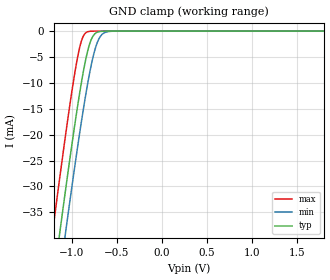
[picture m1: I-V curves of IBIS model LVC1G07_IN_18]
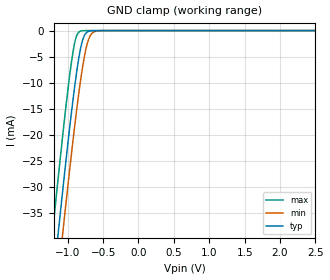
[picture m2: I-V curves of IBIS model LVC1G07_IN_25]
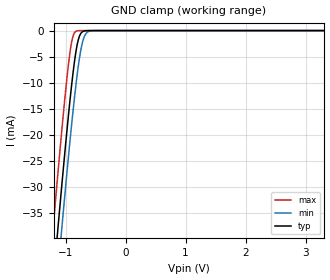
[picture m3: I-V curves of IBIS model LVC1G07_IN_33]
| TEXAS INSTRUMENTS INCORPORATED
| Standard Linear and Logic Group
| IBIS Model of SN74LVC1G07
| SINGLE BUFFER/DRIVER WITH OPEN-DRAIN OUTPUT
| This file contains package information for the following:
|  SON 6-pin (DSF) package as [Component] LVC1G07_DSF
|  SOT 5-pin (DBV) package as [Component] LVC1G07_DBV
|  SOT 5-pin (DCK) package as [Component] LVC1G07_DCK
|  NanoStar WCSP 5-pin (YEP) package as [Component] LVC1G07_YEP
|  NanoFree WCSP 5-pin (YZP) package as [Component] LVC1G07_YZP
|  NanoFree WCSP 5-pin (YZT) package as [Component] LVC1G07_YZT
| This device can be powered at the following Vccs:
|  1.8 volt Vcc
|  2.5 volt Vcc
|  3.3 volt Vcc
|  5 volt Vcc
| This file provides unique models under the [Model Selector] for each Vcc.
| For operation at a specific Vcc, select the appropriate model after each
| [Model Selector] keyword.
[IBIS Ver]   3.2
[Comment char]  |_char
[File Name]   sn74lvc1g07.ibs
[File Rev]   1.4 | d_die
[Date]   03/06/2014
[Source]
| Texas Instruments Incorporated.
| Analog-eLab Design Center, HPA
| 12500 TI Blvd
| Dallas, TX -75243
[Notes]   Revision History:
| The following is an IBIS list for the SN74LVC1G07.
| Please contact sllibis@ti.com with questions and
| comments concerning SLL IBIS models.
| - FILE REV HISTORY
| - 1.2 YEP and YZP packages added on 10/15/2004
| - 1.3 YZT package added on 02/23/2005
| - Power clamp data deleted as there is no power-clamp diode.
| - The slow Rising Waveforms in the LVC1G07_OUT are normal for
|   this open-drain (TPLZ) device.
| - 1.4 DSF package added 03/06/2014.
[Disclaimer]
| Property of Texas Instruments Incorporated.  Unauthorized
| reproduction and/or distribution is strictly prohibited.
| This product is protected under copyright law.
| Created  2002, (C) Copyright  2002, Texas Instruments
| Incorporated, All Rights Reserved
| UNLESS THERE IS A SIGNED, WRITTEN AGREEMENT TO THE
| CONTRARY, TEXAS INSTRUMENTS (TI) IS PROVIDING THE IBIS
| MODELS  AND WITHOUT ANY WARRANTY, EXPRESSED OR
| IMPLIED.  TI assumes no liability for:
|  1) the accuracy of the IBIS models provided to your
|   company;
|  2) the proper functioning of these IBIS Models in your
|   design or for any resulting applications; or
|  3) infringement of patents, copyrights or intellectual
|   property rights resulting from your use of these IBIS
|   models.
| TI provides IBIS Models as a service to our customers.
| You and your company shall not distribute, sell or give
| these models to anyone else without prior written
| permission from TI.
| TI reserves the right to make changes to our products or
| to discontinue any semiconductor product or service
| without notice, and advises our customers to obtain the
| latest version of relevant information to verify, before
| placing orders, that the information being relied on is
| current.
| Please be aware that your receipt and use of the IBIS
| information provided shall serve as acceptance of these
| terms and conditions.  If you do not accept these terms,
| you should return or destroy the IBIS models and any
| other accompanying information immediately.
[Copyright]
(C) Copyright 2014 Texas Instruments Incorporated.All rights reserved.
| Component LVC1G07_DSF 6-pin SON
[Component]   LVC1G07_DSF
[Manufacturer]   Texas Instruments, Inc.
[Package]
|   typ   min   max
R_pkg   0.041145   0.03325   0.04904
L_pkg   0.422435nH  0.33414nH   0.51073nH
C_pkg   0.109645pF  0.10407pF   0.11522pF
[Pin]   signal_name   model_name   R_pin   L_pin   C_pin
1   nc   nc   0.00109   0.02796nH   0.07413pF
2   A   LVC1G07_IN   0.03325   0.33414nH   0.10407pF
3   GND   GND   0.04429   0.45885nH   0.11133pF
4   Y   LVC1G07_OUT   0.04904   0.51073nH   0.11522pF
5   nc   nc   0.00037   0.03788nH   0.07652pF
6   VCC   POWER   0.04377   0.44894nH   0.11085pF
| Component LVC1G07_DBV 5-pin SOT
[Component]   LVC1G07_DBV
[Manufacturer]   Texas Instruments, Inc.
[Package]
|   typ   min   max
R_pkg   2.500e-02   2.100e-02   2.900e-02
L_pkg   1.529e-09   1.312e-09   1.906e-09
C_pkg   1.560e-13   1.100e-13   2.400e-13
[Pin]   signal_name   model_name   R_pin   L_pin   C_pin
1   NC   NC   2.100e-02   1.511e-09   1.440e-13
2   A   LVC1G07_IN   2.300e-02   1.312e-09   1.380e-13
3   GND   GND   2.900e-02   1.906e-09   2.400e-13
4   Y   LVC1G07_OUT   2.600e-02   1.541e-09   1.500e-13
5   VCC   POWER   2.500e-02   1.374e-09   1.100e-13
| Component LVC1G07_DCK 5-pin SOT
[Component]   LVC1G07_DCK
[Manufacturer]   Texas Instruments, Inc.
[Package]
|   typ   min   max
R_pkg   2.000e-02   1.700e-02   2.500e-02
L_pkg   9.980e-10   8.810e-10   1.069e-09
C_pkg   1.460e-13   1.180e-13   2.050e-13
[Pin]   signal_name   model_name   R_pin   L_pin   C_pin
1   NC   NC   1.900e-02   1.069e-09   1.620e-13
2   A   LVC1G07_IN   1.800e-02   8.810e-10   1.210e-13
3   GND   GND   1.700e-02   1.031e-09   2.050e-13
4   Y   LVC1G07_OUT   2.000e-02   9.600e-10   1.240e-13
5   VCC   POWER   2.500e-02   1.049e-09   1.180e-13
| Component LVC1G07_YEP 5-pin NanoStar WCSP
[Component]   LVC1G07_YEP
[Manufacturer]   Texas Instruments, Inc.
[Package]
|   typ   min   max
R_pkg   0.001   0.001   0.001
L_pkg   0.021nH   0.021nH   0.021nH
C_pkg   0.046pF   0.045pF   0.047pF
[Pin]   signal_name   model_name   R_pin   L_pin   C_pin
1   DNU   LVC1G07_IN   0.001   0.021nH   0.046pF
2   A   LVC1G07_IN   0.001   0.021nH   0.047pF
3   GND   GND   0.001   0.021nH   0.046pF
4   Y   LVC1G07_OUT   0.001   0.021nH   0.045pF
5   VCC   POWER   0.001   0.021nH   0.045pF
| Component LVC1G07_YZP 5-pin NanoFree WCSP
[Component]   LVC1G07_YZP
[Manufacturer]   Texas Instruments, Inc.
[Package]
|   typ   min   max
R_pkg   0.001   0.001   0.001
L_pkg   0.021nH   0.021nH   0.021nH
C_pkg   0.046pF   0.045pF   0.047pF
[Pin]   signal_name   model_name   R_pin   L_pin   C_pin
1   DNU   LVC1G07_IN   0.001   0.021nH   0.046pF
2   A   LVC1G07_IN   0.001   0.021nH   0.047pF
3   GND   GND   0.001   0.021nH   0.046pF
4   Y   LVC1G07_OUT   0.001   0.021nH   0.045pF
5   VCC   POWER   0.001   0.021nH   0.045pF
| Component LVC1G07_YZT 5-pin NanoFree WCSP
[Component]   LVC1G07_YZT
[Manufacturer]   Texas Instruments, Inc.
[Package]
|   typ   min   max
R_pkg   0.001   0.001   0.001
L_pkg   0.021nH   0.021nH   0.021nH
C_pkg   0.046pF   0.045pF   0.047pF
[Pin]   signal_name   model_name   R_pin   L_pin   C_pin
1   DNU   LVC1G07_IN   0.001   0.021nH   0.046pF
2   A   LVC1G07_IN   0.001   0.021nH   0.047pF
3   GND   GND   0.001   0.021nH   0.046pF
4   Y   LVC1G07_OUT   0.001   0.021nH   0.045pF
5   VCC   POWER   0.001   0.021nH   0.045pF
| Model LVC1G07_IN
[Model Selector]   LVC1G07_IN
LVC1G07_IN_18   1.8 volt Vcc
LVC1G07_IN_25   2.5 volt Vcc
LVC1G07_IN_33   3.3 volt Vcc
LVC1G07_IN_50   5 volt Vcc
| Model LVC1G07_OUT
[Model Selector]   LVC1G07_OUT
LVC1G07_OUT_18   1.8 volt Vcc
LVC1G07_OUT_25   2.5 volt Vcc
LVC1G07_OUT_33   3.3 volt Vcc
LVC1G07_OUT_50   5 volt Vcc
| Models and submodels in the file (8): LVC1G07_IN_18 (Input), LVC1G07_IN_25 (Input), LVC1G07_IN_33 (Input), LVC1G07_IN_50 (Input), LVC1G07_OUT_18 (Open_drain), LVC1G07_OUT_25 (Open_drain), LVC1G07_OUT_33 (Open_drain), LVC1G07_OUT_50 (Open_drain)
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[Model]   LVC1G07_IN_18
Model_type  Input
Vinl=0.5775
Vinh=1.2675
| variable   typ   min   max
C_comp   3.12pF   2.52pF   4.25pF
[Temperature Range]   40   100   -40
| Ambient temperature   25   85   -40
[Voltage range]   1.8   1.65   1.95
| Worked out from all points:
|   GND clamp passes 1 mA (typ) near -0.77 V on its own axis
[GND Clamp]
| LVC1G07_IN_18
|   Voltage   I(typ)   I(min)   I(max)
-5.5V     -655.2mA   -662.2mA   -646.6mA
-1.215V   -49.6mA    -57.88mA   -38.96mA
-1.135V   -39.07mA   -47.36mA   -28.42mA
-1.075V   -31.35mA   -39.6mA    -20.75mA
-1.055V   -28.82mA   -37.05mA   -18.27mA
-955mV    -16.68mA   -24.66mA   -6.874mA
-885mV    -9.098mA   -16.55mA   -1.486mA
-825mV    -3.922mA   -10.26mA   -137.1uA
-780mV    -1.472mA   -6.227mA   -17.15uA
-715mV    -205.4uA   -2.128mA   -808.5nA
-650mV    -22.01uA   -443.9uA   -37.93nA
1.8V      3.326pA    6.142pA    3.026pA
[Model]   LVC1G07_IN_25
Model_type  Input
Vinl=0.7
Vinh=1.7
| variable   typ   min   max
C_comp   3.14pF   2.51pF   4.31pF
[Temperature Range]   40   100   -40
| Ambient temperature   25   85   -40
[Voltage range]   2.5   2.3   2.7
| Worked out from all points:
|   GND clamp passes 1 mA (typ) near -0.77 V on its own axis
[GND Clamp]
| LVC1G07_IN_25
|   Voltage   I(typ)   I(min)   I(max)
-5.5V     -655.2mA   -662.2mA   -646.6mA
-1.215V   -49.6mA    -57.88mA   -38.96mA
-1.14V    -39.72mA   -48.01mA   -29.07mA
-1.12V    -37.12mA   -45.41mA   -26.48mA
-1.08V    -31.98mA   -40.25mA   -21.38mA
-1.06V    -29.44mA   -37.69mA   -18.89mA
-960mV    -17.26mA   -25.26mA   -7.377mA
-890mV    -9.597mA   -17.1mA    -1.734mA
-785mV    -1.671mA   -6.635mA   -21.67uA
-720mV    -242.5uA   -2.354mA   -1.023uA
-650mV    -22.01uA   -443.9uA   -37.93nA
2.5V      4.713pA    7.577pA    4.389pA
[Model]   LVC1G07_IN_33
Model_type  Input
Vinl=0.8
Vinh=2.0
| variable   typ   min   max
C_comp   3.15pF   2.51pF   4.42pF
[Temperature Range]   40   100   -40
| Ambient temperature   25   85   -40
[Voltage range]   3.3   3   3.6
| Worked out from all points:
|   GND clamp passes 1 mA (typ) near -0.77 V on its own axis
[GND Clamp]
| LVC1G07_IN_33
|   Voltage   I(typ)   I(min)   I(max)
-5.5V     -655.2mA   -662.2mA   -646.6mA
-1.225V   -50.93mA   -59.21mA   -40.3mA
-1.145V   -40.37mA   -48.66mA   -29.72mA
-1.12V    -37.12mA   -45.41mA   -26.48mA
-1.08V    -31.98mA   -40.25mA   -21.38mA
-1.06V    -29.44mA   -37.69mA   -18.89mA
-965mV    -17.84mA   -25.87mA   -7.89mA
-885mV    -9.098mA   -16.55mA   -1.486mA
-780mV    -1.472mA   -6.227mA   -17.15uA
-715mV    -205.4uA   -2.128mA   -808.5nA
-640mV    -15.53uA   -338.1uA   -23.69nA
3.3V      6.304pA    9.258pA    5.93pA
